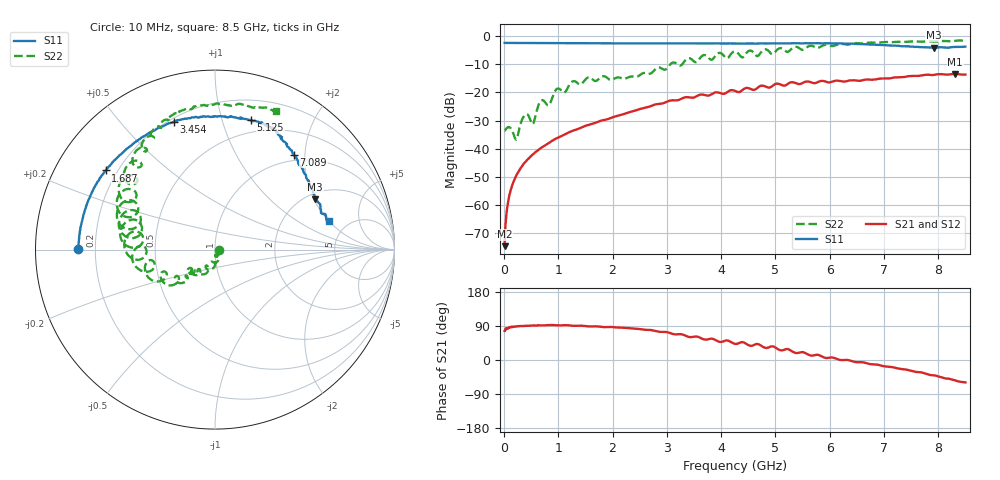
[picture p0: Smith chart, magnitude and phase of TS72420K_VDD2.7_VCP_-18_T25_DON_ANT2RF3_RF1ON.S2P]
!Agilent Technologies,E5071C,MY46417908,A.11.23
!Date: Thu Oct 03 16:40:43 2019
!Data & Calibration Information:
!Freq	S11:SOLT2(ON)	S21:SOLT2(ON)	S12:SOLT2(ON)	S22:SOLT2(ON)
!PortZ  Port1:50+j0  Port2:50+j0
!Above PortZ is port z conversion or system Z0 setting when saving the data.
!When reading, reference impedance value at option line is always used.
# Hz S dB R 50
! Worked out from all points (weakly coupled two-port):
!   1601 points, 10 MHz to 8.5 GHz, reference 50 ohm
!   highest |S21| = -13.40 dB at 8.314 GHz (marker M1); lowest = -74.7 dB at 10 MHz (marker M2)
!   lowest |S11| = -4.1 dB at 7.916 GHz (marker M3), VSWR 4.32, Z = 111 + j102 ohm
!   |S11| at or under -10 dB: nowhere
!   |S22| runs from -36.8 to -1.5 dB; largest |S21 - S12| = 0.0025
!   S11 on the Smith chart (normalised r, x): 10 MHz: 0.13, +0.00; 1.687 GHz: 0.16, +0.32; 3.454 GHz: 0.22, +0.70; 5.125 GHz: 0.38, +1.24; 7.089 GHz: 0.89, +1.78; 8.5 GHz: 3.59, +2.02
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1e7  -2.35 179.8  -74.71 76.6  -74.55 83.4  -33.61 -0.7
6.836875e7  -2.37 178.4  -59.63 83.0  -59.71 84.2  -32.38 -19.8
1.16125e8  -2.37 177.2  -55.15 86.3  -55.13 86.7  -32.59 -38.3
2.275562e8  -2.39 174.5  -49.48 88.5  -49.46 88.6  -36.68 -44.2
3.336812e8  -2.39 172.2  -46.15 89.7  -46.08 89.7  -29.51 -40.6
4.185812e8  -2.40 170.3  -44.16 90.1  -44.18 90.4  -27.70 -76.9
5.300125e8  -2.42 167.8  -42.07 90.8  -42.06 90.7  -31.33 -78.2
6.67975e8  -2.41 164.8  -39.89 91.4  -39.90 91.5  -23.15 -81.1
8.271625e8  -2.42 161.2  -37.97 92.2  -37.96 92.2  -24.54 -97.4
9.757375e8  -2.42 158.1  -36.25 91.5  -36.24 91.5  -18.68 -105.1
1.426769e9  -2.46 149.1  -32.46 90.4  -32.46 90.4  -16.93 -125.1
1.686775e9  -2.47 144.1  -30.77 88.9  -30.77 88.9  -15.93 -136.0
2.843538e9  -2.55 120.2  -24.08 74.7  -24.08 74.7  -11.09 -140.5
3.453756e9  -2.52 108.0  -21.87 60.4  -21.86 60.4  -8.18 -169.0
4.255e9  -2.60 92.5  -19.45 42.5  -19.43 42.4  -5.42 168.5
4.992569e9  -2.50 79.1  -17.03 33.6  -16.97 33.6  -5.63 159.7
5.125225e9  -2.52 74.5  -17.45 25.5  -17.38 25.5  -4.37 146.8
5.671769e9  -2.51 67.3  -16.50 11.6  -16.45 11.9  -3.42 133.6
7.088538e9  -3.25 50.3  -15.02 -17.9  -14.96 -17.6  -2.08 105.6
7.916312e9  -4.10 26.7  -13.78 -40.5  -13.81 -40.5  -1.86 84.8
8.314281e9  -3.79 16.8  -13.40 -53.8  -13.40 -54.4  -1.61 72.5
8.5e9  -3.68 14.2  -13.62 -59.1  -13.66 -59.2  -1.49 66.2
